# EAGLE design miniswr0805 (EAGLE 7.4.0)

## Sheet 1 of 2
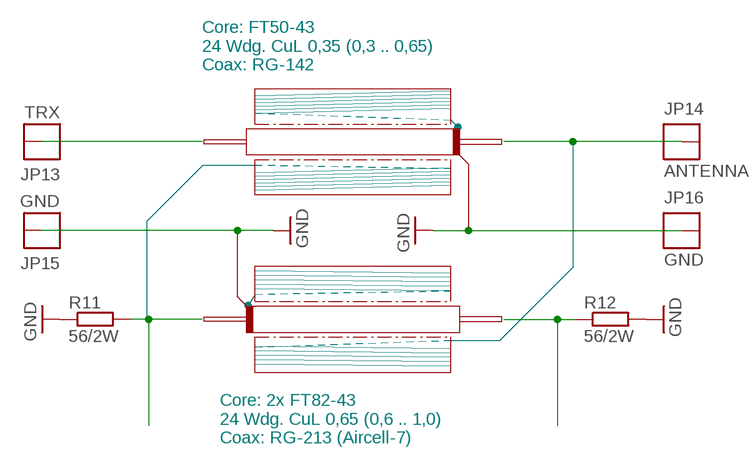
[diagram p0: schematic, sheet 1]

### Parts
JP13  TRX  THICKPINSQUARE  [THICKPIN]
JP14  ANTENNA  THICKPINSQUARE  [THICKPIN]
JP15  GND  THICKPINSQUARE  [THICKPIN]
JP16  GND  THICKPINSQUARE  [THICKPIN]
R11  56/2W  R-EU_0411/12  [0411/12]
R12  56/2W  R-EU_0411/12  [0411/12]

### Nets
GND: JP15.1 JP16.1 R11.1 R12.2 ; also sheet 2
N$15: JP14.1
N$16: JP13.1
PWR: R11.2 ; also sheet 2
SWR: R12.1 ; also sheet 2

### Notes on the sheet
- Core: FT50-43
  24 Wdg. CuL 0,35 (0,3 .. 0,65)
  Coax: RG-142
- Core: 2x FT82-43
  24 Wdg. CuL 0,65 (0,6 .. 1,0)
  Coax: RG-213 (Aircell-7)

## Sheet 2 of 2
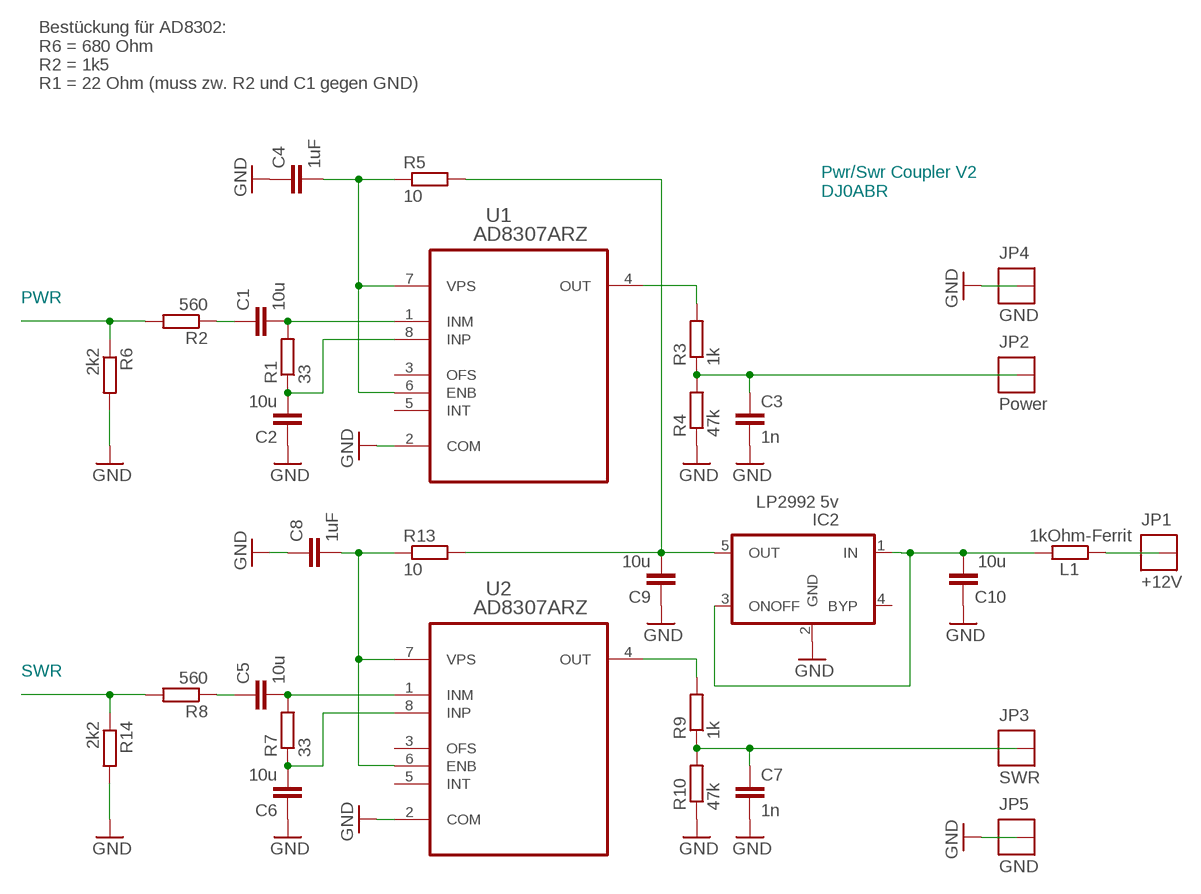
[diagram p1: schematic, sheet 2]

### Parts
C1  10u  C-EUC0805  [C0805]
C2  10u  C-EUC0805  [C0805]
C3  1n  C-EUC0805  [C0805]
C4  1uF  C-EUC0805  [C0805]
C5  10u  C-EUC0805  [C0805]
C6  10u  C-EUC0805  [C0805]
C7  1n  C-EUC0805  [C0805]
C8  1uF  C-EUC0805  [C0805]
C9  10u  C-EUC0805  [C0805]
C10  10u  C-EUC0805  [C0805]
IC2  LP2992 5v  UREG5  [SOT23-5]
JP1  +12V  THICKPINSQUARE  [THICKPIN]
JP2  Power  THICKPINSQUARE  [THICKPIN]
JP3  SWR  THICKPINSQUARE  [THICKPIN]
JP4  GND  THICKPINSQUARE  [THICKPIN]
JP5  GND  THICKPINSQUARE  [THICKPIN]
L1  1kOhm-Ferrit  R-EU_R0805  [R0805]
R1  33  R-EU_R0805  [R0805]
R2  560  R-EU_R0805  [R0805]
R3  1k  R-EU_R0805  [R0805]
R4  47k  R-EU_R0805  [R0805]
R5  10  R-EU_R0805  [R0805]
R6  2k2  R-EU_R0805  [R0805]
R7  33  R-EU_R0805  [R0805]
R8  560  R-EU_R0805  [R0805]
R9  1k  R-EU_R0805  [R0805]
R10  47k  R-EU_R0805  [R0805]
R13  10  R-EU_R0805  [R0805]
R14  2k2  R-EU_R0805  [R0805]
U1  AD8307ARZ  [SOIC127P600X175-8N]
U2  AD8307ARZ  [SOIC127P600X175-8N]

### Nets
GND: C2.1 C3.2 C4.1 C6.1 C7.2 C8.1 C9.1 C10.1 IC2.2(GND) JP4.1 JP5.1 R4.1 R6.2 R10.1 R14.2 U1.2(COM) U2.2(COM) ; also sheet 1
N$1: C1.2 R1.2 U1.1(INM)
N$2: C2.2 R1.1 U1.8(INP)
N$3: C4.2 R5.1 U1.6(ENB) U1.7(VPS)
N$4: C1.1 R2.1
N$5: C3.1 JP2.1 R3.1 R4.2
N$6: R3.2 U1.4(OUT)
N$7: C9.2 IC2.5(OUT) R5.2 R13.2
N$8: JP1.1 L1.1
N$9: C5.2 R7.2 U2.1(INM)
N$10: C6.2 R7.1 U2.8(INP)
N$11: C8.2 R13.1 U2.6(ENB) U2.7(VPS)
N$12: C5.1 R8.1
N$17: C7.1 JP3.1 R9.1 R10.2
N$18: R9.2 U2.4(OUT)
N$20: C10.2 IC2.1(IN) IC2.3(ONOFF) L1.2
PWR: R2.2 R6.1 ; also sheet 1
SWR: R8.2 R14.1 ; also sheet 1
Unconnected: U1.3(OFS) U1.5(INT) U2.3(OFS) U2.5(INT)

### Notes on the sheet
- Bestückung für AD8302:
  R6 = 680 Ohm
  R2 = 1k5
  R1 = 22 Ohm (muss zw. R2 und C1 gegen GND)
- Pwr/Swr Coupler V2
  DJ0ABR
- PWR
- SWR

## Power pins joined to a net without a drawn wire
BYP: IC2.4(BYP)

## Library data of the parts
C1-C10 = rcl:C-EU: CAPACITOR, European symbol
IC2 = km:UREG5
JP1-JP5 JP13-JP16 = km:THICKPIN
L1 R1-R14 = rcl:R-EU_: RESISTOR, European symbol
U1 U2 = ad8307:AD8307ARZ: Low Cost, DC to 500 MHz, 92 dB Logarithmic Amplifier; MPN: AD8307ARZ; OC_FARNELL: 1661041; OC_NEWARK: 59K6564; PACKAGE: SOIC-8; SUPPLIER: Analog Devices

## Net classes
1 dick: width 0.61 mm

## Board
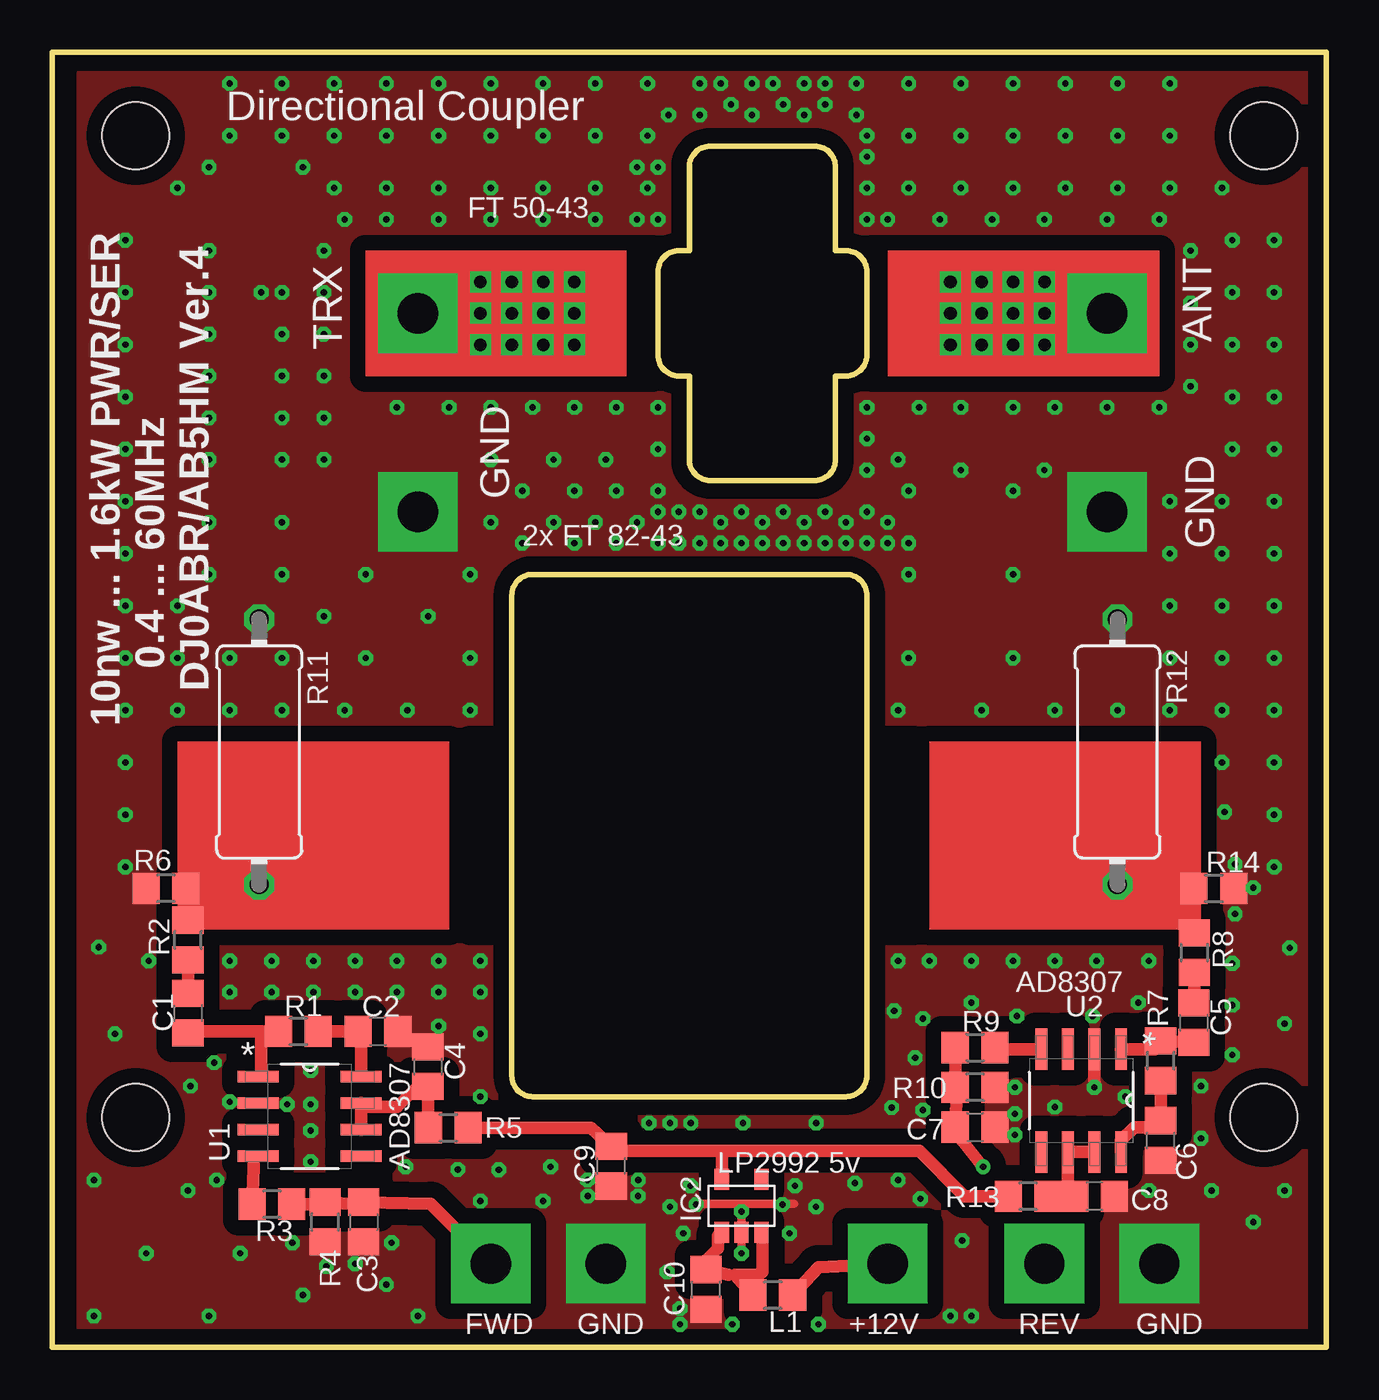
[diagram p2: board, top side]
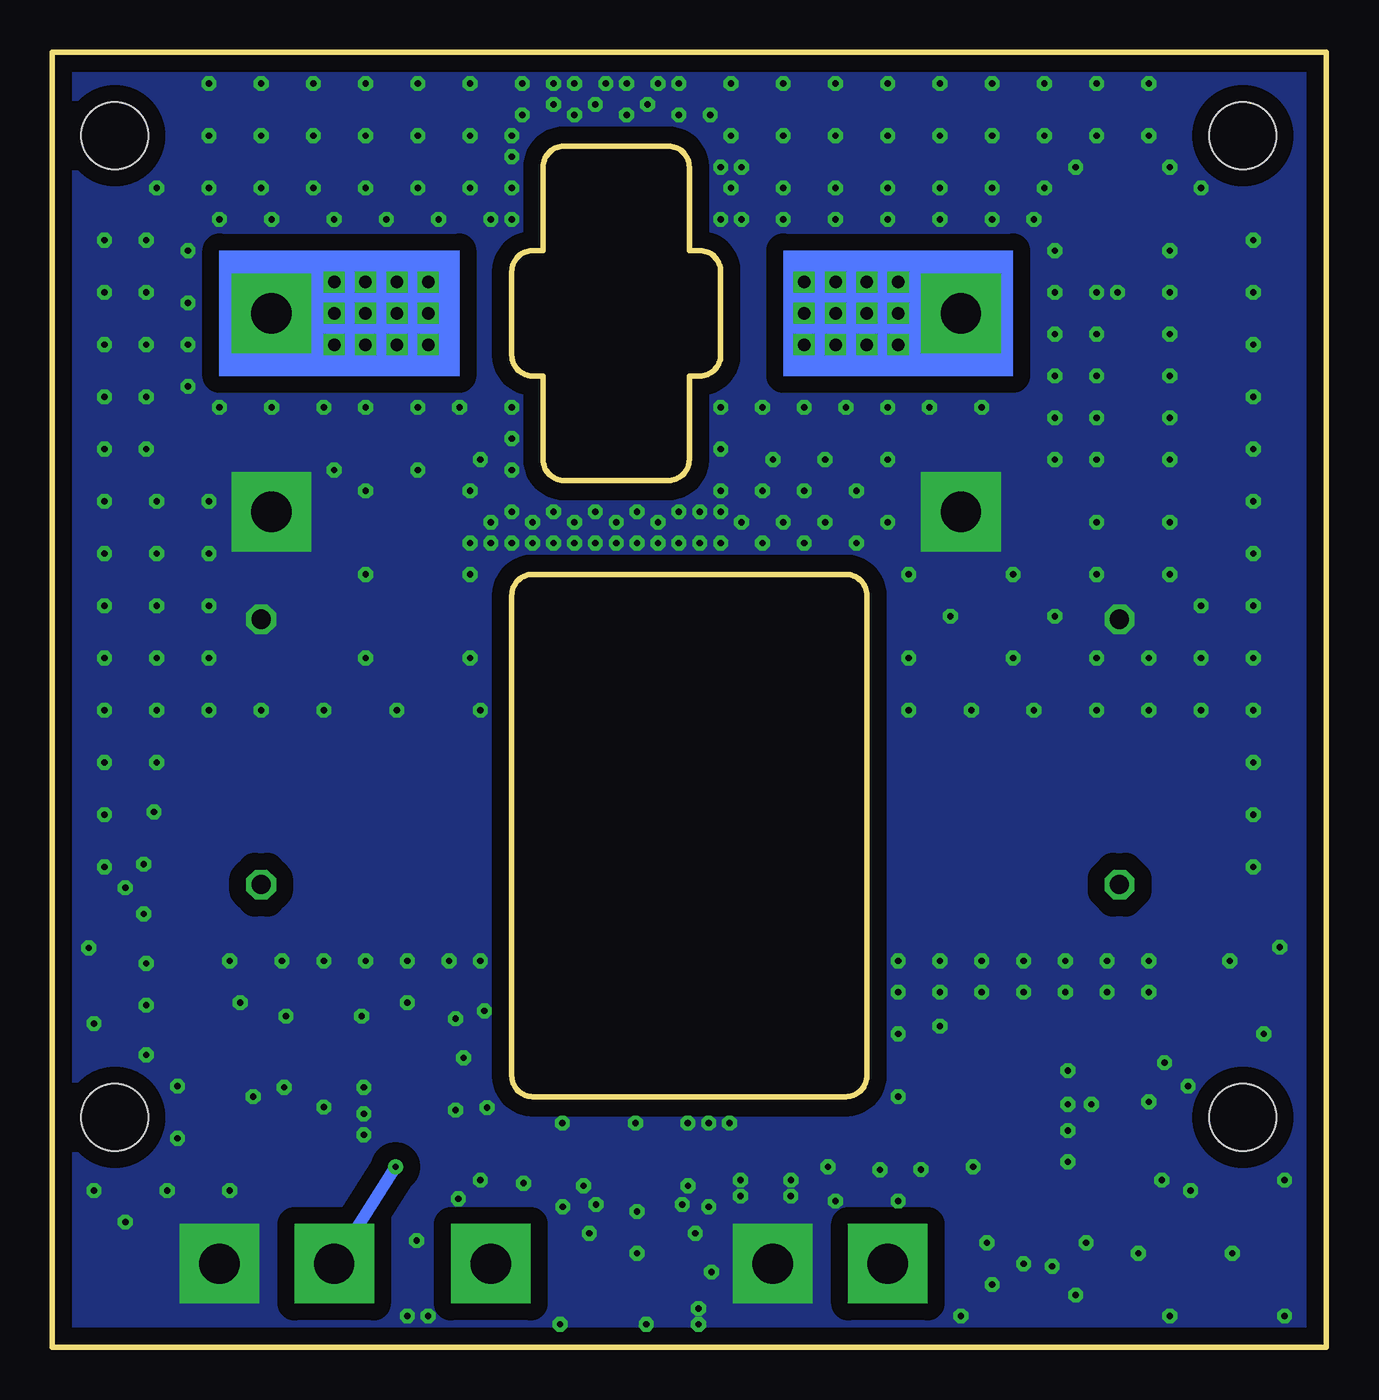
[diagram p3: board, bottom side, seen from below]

Size 61 x 62 mm. Coordinates in mm from the lower left corner, seen from the top.
Outline: 0,62 61,62 61,0 0,0 0,62
Outline: 31.5,57.5 36.5,57.5 arc-90 37.5,56.5 37.5,52.5 38,52.5 arc-90 39,51.5 39,47.5 arc-90 38,46.5 37.5,46.5 37.5,42.5 arc-90 36.5,41.5 31.5,41.5 arc-90 30.5,42.5 30.5,46.5 30,46.5 arc-90 29,47.5 29,51.5 arc-90 30,52.5 30.5,52.5 30.5,56.5 arc-90 31.5,57.5
Outline: 39,36 39,13 arc-90 38,12 23,12 arc-90 22,13 22,36 arc-90 23,37 38,37 arc-90 39,36
Copper layers (1*16): Top 0.035mm / dielectric 1.5mm / Bottom 0.035mm
Design rules "miniswr *": minimum track width 8mil, minimum drill 0.3mm, track to track 12mil, track to pad 12mil, pad to pad 0.205mm, via to via 12mil, smd to smd 0mil, copper to edge 20mil, drill to drill 8mil, minimum pad ring 10mil, minimum via ring 8mil, stop-mask expansion 4mil, vias tented up to drill 1mm, thermal gap 10mil
Holes 3.2 mm at 4,11 58,11 4,58 58,58
tRestrict: area 20,20 to 21,29; area 40,20 to 41.2,29; area 28,46.5 to 28.8,52.5; area 39.2,46.5 to 40,52.5

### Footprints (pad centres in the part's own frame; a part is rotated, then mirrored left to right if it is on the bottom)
C0805 = smd 1.3 x 1.5: 1 -0.95,0; 2 0.95,0
SOT23-5 = smd 0.686 x 0.991: 1 -0.953,0; 2 0,0; 3 0.953,0; 4 0.953,2.54; 5 -0.953,2.54
THICKPIN = drill 1.93 pad 3.81 square: 1 0,0
R0805 = smd 1.3 x 1.5: 1 -0.95,0; 2 0.95,0
0411/12 = drill 0.914 octagon: 1 -6.35,0; 2 6.35,0
SOIC127P600X175-8N = smd 1.981 x 0.559: 1 -2.464,1.905; 2 -2.464,0.635; 3 -2.464,-0.635; 4 -2.464,-1.905; 5 2.464,-1.905; 6 2.464,-0.635; 7 2.464,0.635; 8 2.464,1.905

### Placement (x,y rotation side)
C1  6.5,16 270 top
C2  15.6,15.12 180 top
C3  14.91,6 270 top
C4  17.98,13.44 270 top
C5  54.65,15.54 270 top
C6  53.07,9.9 90 top
C7  44.18,10.54 0 top
C8  49.9,7.23 180 top
C9  26.76,8.66 90 top
C10  31.3,2.77 90 top
IC2  33,5.5 0 top
JP1  40,4 0 top
JP2  21,4 0 top
JP3  47.5,4 0 top
JP4  26.5,4 0 top
JP5  53,4 0 top
JP13  17.5,49.5 0 top
JP14  50.5,49.5 0 top
JP15  17.5,40 0 top
JP16  50.5,40 0 top
L1  34.5,2.5 180 top
R1  11.79,15.12 180 top
R2  6.5,19.5 90 top
R3  10.52,6.86 180 top
R4  13.06,6 90 top
R5  18.96,10.51 0 top
R6  5.45,21.97 180 top
R7  53.07,13.71 90 top
R8  54.68,18.89 90 top
R9  44.18,14.35 0 top
R10  44.18,12.45 180 top
R11  9.9,28.5 270 top
R12  51,28.5 90 top
R13  46.72,7.23 180 top
R14  55.61,21.97 0 top
U1  12.32,11.05 0 top
U2  49.26,11.81 270 top

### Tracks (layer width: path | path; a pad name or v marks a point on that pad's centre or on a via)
GND  (via drill 0.3)
  Top 0.406: v33,4.5 IC2.2 v33,6.5 33,6.88 | 35.5,6.88 33,6.88 | 31,6.88 33,6.88
  Top 0.61: v49.9,12.45 U2.2
  other vias: 20,37 20,33 20,30.5 17,30.5 15,33 15,37 11,37 11,33 14,30.5 18.5,18.5 41,41 41,37 41,33 40.5,30.5 44.5,30.5 46,33 46,37 46,41 48,30.5 46.09,12.45 46.09,11.18 36.56,6.73 8.5,60.5 11,60.5 13.5,60.5 16,60.5 18.5,60.5 21,60.5 23.5,60.5 26,60.5 28.5,60.5 31,60.5 33.5,60.5 36,60.5 38.5,60.5 41,60.5 43.5,60.5 46,60.5 48.5,60.5 51,60.5 53.5,60.5 8.5,58 7.5,56.5 12,56.5 13.5,55.5 16,55.5 18.5,55.5 41,55.5 43.5,55.5 46,55.5 48.5,55.5 51,55.5 53.5,55.5 53.5,58 41,58 18.5,58 3.5,53 3.5,50.5 3.5,48 3.5,45.5 3.5,43 3.5,40.5 3.5,38 3.5,35.5 3.5,33 3.5,30.5 3.5,28 3.5,25.5 3.5,23 58.5,53 58.5,50.5 58.5,48 58.5,45.5 58.5,43 58.5,40.5 58.5,38 58.5,35.5 58.5,33 58.5,30.5 58.5,28 58.5,25.5 58.5,23 56,28 56,30.5 56,33 56,35.5 56,38 56,40.5 53.5,40.5 53.5,38 53.5,35.5 53.5,33 53.5,30.5 52.5,18.5 51,30.5 6,35.5 6,33 6,30.5 16.5,18.5 20.5,18.5 8.5,30.5 8.5,33 11,30.5 56,55.5 6,55.5 11,58 13.5,58 16,58 43.5,58 46,58 48.5,58 51,58 23.5,7 14.5,4 16,3 19.41,8.51 23.86,8.63 25.63,8 25.64,7.24 28.05,7.24 28.05,8 29.57,6.73 30.21,5.46 35.29,5.46 16.25,5 11.5,5 21.38,8.5 20.5,7 17.5,1.5 3,15 6.5,7.5 2,8 2,1.5 7.5,1.5 59,7.5 55.5,7.5 52.5,7.5 55,10 56.5,14 59,15.5 55,12.5 51.38,12 48,11.5 57.5,6 43,1.5 44,1.5 30.84,6.83 34.96,6.83 41.56,7.11 40.5,8 35.56,7.73 30.56,7.73 30.06,1.85 29.43,3.6 32.56,1.1 36.69,1.1 30.06,1.1 40.19,11.48 41.69,11.36 40.31,16.11 46.19,15.86 49.81,15.86 41.69,15.73 41.31,13.86 38.44,7.86 21,58 23.5,58 26,58 28.5,58 21,55.5 23.5,55.5 26,55.5 28.5,55.5 22.5,41 25,41 27,41 29,41 29,45 29,43 26,54 23.5,54 21,54 18.5,54 13,42.5 22.5,38.5 25,38.5 27,38.5 29,38.5 31,38.5 33,38.5 35,38.5 37,38.5 39,38.5 41,38.5 31,40 33,40 35,40 37,40 39,40 39,42 39,43.5 39,45 40.5,42.5 43.5,42 47.5,42 32,39.5 34,39.5 36,39.5 38,39.5 40,39.5 32,38.5 34,38.5 36,38.5 38,38.5 40,38.5 30,38.5 30,40 29,40 28,39.5 26,39.5 24,39.5 21,39.5 29.5,59 31,59 33.5,59 36,59 38.5,59 39,58 37,59.5 35,59.5 32.5,59.5 32,60.5 34.5,60.5 37,60.5 39,57 39,55.5 39,54 40,54 29,54 28,54 29,56.5 28,56.5 56.5,53 56.5,50.5 56.5,48 56.5,45.5 56.5,43 21,42.5 24,42.5 26.5,42.5 13,44.5 13,46.5 13,48.5 13,50.5 13,52.5 14,54 16,54 10,50.5 11,50.5 11,48.5 11,46.5 11,44.5 11,42.5 11,39.5 7.5,52.5 7.5,50.5 7.5,48.5 7.5,46.5 7.5,44.5 7.5,42.5 7.5,39.5 7.5,37 30.57,10.73 29.57,10.73 28.57,10.73 27,45 25,45 23,45 21,45 19,45 16.5,45 41.5,45 43.5,45 46,45 48,45 50.5,45 53,45 54.5,46 54.5,48 54.5,50 54.5,52.5 53,54 50.5,54 47.5,54 45,54 42.5,54 33.08,10.73 36.58,10.73 43.56,5.11 4.5,4.5 9,4.5 12,2.5 14.5,18.5 12.5,18.5 10.5,18.5 8.5,18.5 10.5,17 12.5,17 14.5,17 16.5,17 18.5,17 20.5,17 20.5,15 20.5,12 18,35 13,35 50,18.5 48,18.5 46,18.5 44,18.5 42,18.5 40.5,18.5 52,16.5 44,16.5 6.62,12.5 4.62,18.5 8.5,17 8.5,11.75 11.25,11.62 12.38,13.25 12.38,11.62 12.38,10.38 12.38,8.88 18.5,15.38 13.12,3.88 7.88,8 7.75,13.62 16.91,8.63 56.5,18.38 56.5,16.38 56.62,20.75 57.5,22 56.62,23.12 56.12,25.62 59.25,19.12 46.09,10.18 2.23,19.15
  pour Top (isolate 0.75, no thermals): 1.36,61 60,61 60,0.74 1.36,0.74
  pour Bottom (isolate 0.813, no thermals): 1,61.34 60.69,61.34 60.69,0.38 1,0.38
N$1
  Top 0.61: C1.2 6.5,15.12 10,15.12 | 10,15.12 R1.2 | U1.1 10,13.1 10,15.12
N$2
  Top 0.61: R1.1 C2.2 14.79,15.05 U1.8
N$3
  Top 0.61: U1.6 U1.7 14.98,11.5 16.5,11.5 17.56,12.56 C4.2 17.98,10.63 R5.1
N$4
  Top 0.61: R2.1 C1.1
N$5
  Top 0.406: 13.06,6.86 R4.2 | 14.66,6.85 C3.1
  Top 0.61: R3.1 13.06,6.86 | R4.2 14.66,6.85 | C3.1 18.12,6.88 JP2.1
N$6
  Top 0.406: U1.4 9.67,9.15
  Top 0.61: 9.67,9.15 R3.2
N$7
  Top 0.61: C9.2 27.01,9.29 | 32.05,9.4 27.12,9.4 arc90 C9.2 | R13.2 43.68,7.23 41.51,9.4 32.05,9.4 | IC2.5 32.05,9.4 | C9.2 25.79,10.51 R5.2
N$8
  Top 0.61: L1.1 36.68,3.83 JP1.1
N$9
  Top 0.61: U2.1 52.78,14.27 R7.2 53.17,14.67 C5.2
N$10
  Top 0.61: R7.1 C6.2 52.83,10.54 51.8,10.54 51.16,9.9 U2.8
N$11
  Top 0.61: U2.7 U2.6 48.62,7.12 C8.2 R13.1
N$12
  Top 0.61: C5.1 54.68,16.45 R8.1
N$13  (via drill 0.6)
  other vias: 20.5,51
N$14  (via drill 0.6)
  other vias: 22,51
N$17  (via drill 0.3)
  Top 0.61: R9.1 R10.2 43.3,12.42 C7.1 43.55,9.9 v44.56,8.63
  Bottom 0.61: v44.56,8.63 JP3.1
N$18
  Top 0.61: R9.2 45.11,14.27 U2.4
N$19  (via drill 0.6)
  other vias: 23.5,51
N$20
  Top 0.406: IC2.1 31.88,5.33 | 32.68,3.47 32.38,3.47 | IC2.3 34,5.45
  Top 0.61: 31.88,5.33 31.88,4.75 31.3,4.17 C10.2 32.38,3.47 | L1.2 32.68,3.47 33.84,3.47 34,3.62 34,5.45
N$21  (via drill 0.6)
  other vias: 25,51
N$23  (via drill 0.6)
  other vias: 20.5,48
N$24  (via drill 0.6)
  other vias: 22,48
N$25  (via drill 0.6)
  other vias: 23.5,48
N$26  (via drill 0.6)
  other vias: 25,48
N$28  (via drill 0.6)
  other vias: 47.5,51
N$29  (via drill 0.6)
  other vias: 46,51
N$30  (via drill 0.6)
  other vias: 44.5,51
N$31  (via drill 0.6)
  other vias: 43,51
N$33  (via drill 0.6)
  other vias: 47.5,48
N$34  (via drill 0.6)
  other vias: 46,48
N$35  (via drill 0.6)
  other vias: 44.5,48
N$36  (via drill 0.6)
  other vias: 43,48
N$38  (via drill 0.6)
  other vias: 47.5,49.5
N$39  (via drill 0.6)
  other vias: 46,49.5
N$40  (via drill 0.6)
  other vias: 44.5,49.5
N$41  (via drill 0.6)
  other vias: 43,49.5
N$43  (via drill 0.6)
  other vias: 20.5,49.5
N$44  (via drill 0.6)
  other vias: 22,49.5
N$45  (via drill 0.6)
  other vias: 23.5,49.5
N$46  (via drill 0.6)
  other vias: 25,49.5
PWR
  Top 0.254: R6.1 8.35,22.14 8.35,22.5
  Top 0.406: R2.2 R6.1
  Top 3.81: R11.2 8.35,22.5
SWR
  Top 0.254: R14.1 51,21.97 R12.1
  Top 0.406: R8.2 R14.1
  Top 3.81: 44.85,22.15 R12.1
(copper drawn outside any net)
  shapes: Bottom area x2, Top area x4

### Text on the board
tNames: Directional Coupler | FT 50-43 | TRX | ANT | GND | 2x FT 82-43 | GND | 10nw ... 1.6kW PWR/SER / 0.4 ... 60MHz / DJ0ABR/AB5HM Ver.4 | AD8307 | AD8307 | FWD | GND | +12V | REV | GND
tValues: LP2992 5v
